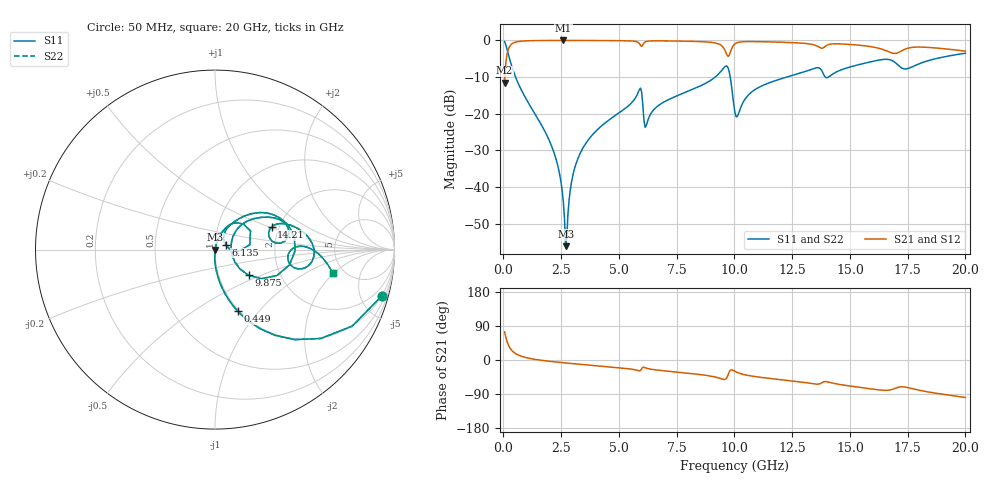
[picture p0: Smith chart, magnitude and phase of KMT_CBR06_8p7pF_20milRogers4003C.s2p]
! Data measured by Modelithics Inc. support@modelithics.com 813-866-6335
! KEMET CBR0603 8.7pF, Pad Width= 0.851mm, Pad Length= 0.64mm, Pad Gap= 0.62mm, 20mil Rogers 4003C substrate Data, January 2022
# hz S ma R 50
! 2 Port Network Data from SP1.SP block
! freq  magS11  angS11  magS21  angS21  magS12  angS12  magS22  angS22
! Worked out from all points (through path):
!   401 points, 50 MHz to 20 GHz, reference 50 ohm
!   highest |S21| = -0.01 dB at 2.594 GHz (marker M1); lowest = -11.5 dB at 50 MHz (marker M2)
!   group delay of S21, straight-line fit = 14.5 ps
!   lowest |S11| = -56.1 dB at 2.693 GHz (marker M3), VSWR 1.00, Z = 50.1 - j0.107 ohm
!   |S11| at or under -10 dB: 524.7 MHz to 9.166 GHz (8.641 GHz wide, 178 % of centre); 9.818 GHz to 12.27 GHz (2.448 GHz wide, 22.2 % of centre); 13.94 GHz to 14.07 GHz (132.3 MHz wide, 0.944 % of centre)
!   |S22| runs from -56.1 to -0.3 dB; largest |S21 - S12| = 0
!   S11 on the Smith chart (normalised r, x): 50 MHz: 0.98, -7.19; 449 MHz: 0.98, -0.78; 6.135 GHz: 1.12, +0.06; 9.875 GHz: 1.39, -0.42; 14.21 GHz: 1.83, +0.52; 20 GHz: 4.07, -1.94
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5e7  0.964 -15.6  0.2656 74.4  0.2656 74.4  0.964 -15.6
2.495e8  0.5847 -54.9  0.8104 35.1  0.8104 35.1  0.5847 -54.9
4.49e8  0.3659 -69.7  0.9298 20.2  0.9298 20.2  0.3659 -69.7
2.14475e9  0.03228 -92.4  0.9982 -4.4  0.9982 -4.4  0.03228 -92.4
2.444e9  0.01432 -91.4  0.9986 -6.3  0.9986 -6.3  0.01432 -91.4
2.593625e9  0.006233 -85.6  0.9986 -7.2  0.9986 -7.2  0.006233 -85.6
2.693375e9  0.001562 -43.2  0.9986 -7.8  0.9986 -7.8  0.001562 -43.2
3.0425e9  0.01619 75.4  0.9984 -9.8  0.9984 -9.8  0.01619 75.4
3.391625e9  0.03192 75.7  0.9979 -11.7  0.9979 -11.7  0.03192 75.7
5.885375e9  0.2134 41.5  0.9072 -28.7  0.9072 -28.7  0.2134 41.5
6.13475e9  0.06505 25.4  0.9534 -20.5  0.9534 -20.5  0.06505 25.4
6.73325e9  0.1311 60.6  0.9858 -27.1  0.9858 -27.1  0.1311 60.6
9.227e9  0.3285 38.9  0.914 -45.8  0.914 -45.8  0.3285 38.9
9.626e9  0.4471 8.5  0.6922 -50.3  0.6922 -50.3  0.4471 8.5
9.875375e9  0.2363 -37.4  0.7671 -25.8  0.7671 -25.8  0.2363 -37.4
1.0025e10  0.1024 -19.7  0.8988 -30.0  0.8988 -30.0  0.1024 -19.7
1.087288e10  0.2116 42.8  0.9636 -43.5  0.9636 -43.5  0.2116 42.8
1.336662e10  0.4058 23.2  0.8817 -62.3  0.8817 -62.3  0.4058 23.2
1.42145e10  0.3402 21.8  0.8951 -60.5  0.8951 -60.5  0.3402 21.8
1.670825e10  0.5471 -6.0  0.694 -79.4  0.694 -79.4  0.5471 -6.0
1.74065e10  0.4078 -5.2  0.7637 -71.6  0.7637 -71.6  0.4078 -5.2
2e10  0.669 -11.3  0.7137 -98.9  0.7137 -98.9  0.669 -11.3
